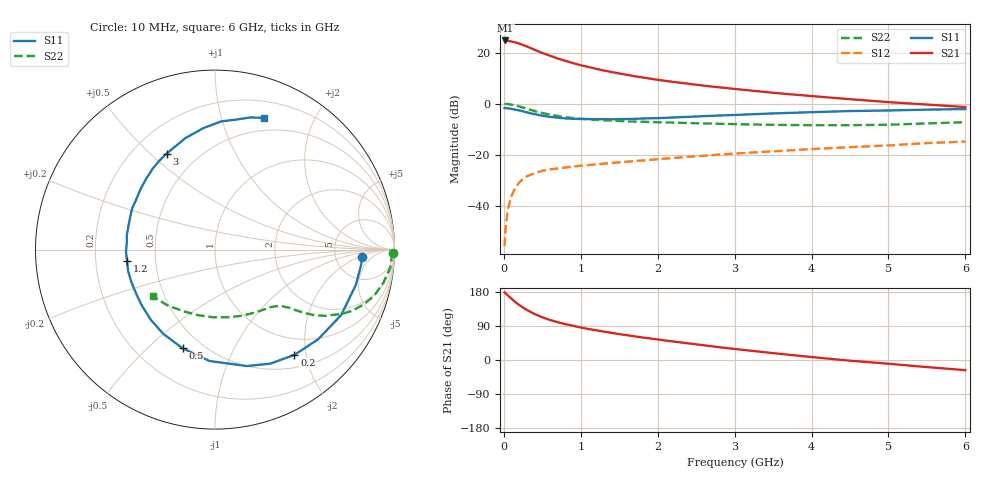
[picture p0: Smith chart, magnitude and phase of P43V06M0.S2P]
! SIEMENS Small Signal Semiconductors
! BFP182
! Si NPN RF Bipolar Junction Transistor in SOT143
! VCE = 3 V  IC = 6 mA
! Common Emitter S-Parameters:  March  1996
# GHz  S  MA  R  50
!  f  S11  S21  S12  S22
! GHz  MAG  ANG  MAG  ANG  MAG  ANG  MAG  ANG
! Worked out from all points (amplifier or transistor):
!   36 points, 10 MHz to 6 GHz, reference 50 ohm
!   highest |S21| = 24.8 dB at 20 MHz (marker M1)
!   |S21| within 3 dB of that: start of sweep to 349.4 MHz
!   unconditionally stable (mu >= 1): 1.477 GHz to 5.459 GHz
!   at 250 MHz: K = 0.24, MSG = 26.2 dB, |S12| = -29.5 dB
!   at 1.4 GHz: K = 0.98, MSG = 17.9 dB, |S12| = -23.3 dB
!   at 6 GHz: K = 0.93, MSG = 6.8 dB, |S12| = -14.9 dB
!   lowest NFmin = 1.25 dB at 450 MHz
!   S11 on the Smith chart (normalised r, x): 10 MHz: 9.55, -2.24; 200 MHz: 0.70, -1.79; 500 MHz: 0.39, -0.65; 1.2 GHz: 0.34, -0.05; 3 GHz: 0.34, +0.56; 6 GHz: 0.36, +1.38
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0.01  0.8195 -2.7  17.16 178.2  0.0016 78.4  0.9892 -1.1
0.02  0.8191 -5.7  17.35 176.6  0.0032 89.8  0.9848 -2.3
0.05  0.809 -14.1  17.15 170.6  0.0083 85.6  0.9822 -5.8
0.1  0.792 -27.4  16.53 161.7  0.0155 75.0  0.9556 -11.2
0.15  0.7617 -41.0  15.91 152.9  0.0224 69.1  0.9234 -16.2
0.2  0.7346 -53.0  15.06 145.1  0.0284 64.0  0.881 -20.4
0.25  0.7064 -64.1  14.07 138.1  0.0334 58.9  0.8376 -24.0
0.3  0.6724 -74.8  13.21 132.0  0.0377 55.3  0.7919 -26.9
0.4  0.6212 -92.9  11.39 121.2  0.0432 48.7  0.715 -31.1
0.5  0.5783 -108.2  9.843 112.7  0.0482 44.6  0.6555 -33.7
0.6  0.551 -121.4  8.719 105.6  0.0513 41.2  0.6086 -35.4
0.7  0.53 -132.5  7.665 99.8  0.0535 39.8  0.5709 -36.6
0.8  0.5131 -142.6  6.92 94.5  0.0558 38.3  0.5426 -37.6
1.1  0.4985 -166.2  5.229 81.8  0.0624 36.6  0.4922 -40.0
1.2  0.4945 -172.9  4.816 78.4  0.0642 36.2  0.4808 -41.0
1.7  0.5033 161.0  3.445 62.5  0.0746 36.2  0.4439 -46.4
2.2  0.5344 141.0  2.671 48.8  0.0857 35.9  0.4241 -53.6
3  0.5992 116.7  1.945 29.2  0.1048 33.4  0.3969 -68.5
3.5  0.6426 104.9  1.633 18.1  0.116 30.9  0.3835 -79.5
4.5  0.7153 87.2  1.222 -1.8  0.14 25.3  0.3775 -104.6
5.5  0.7623 75.0  0.959 -18.7  0.1682 19.5  0.4091 -130.8
6  0.7835 69.4  0.858 -26.8  0.1801 15.0  0.4332 -143.3
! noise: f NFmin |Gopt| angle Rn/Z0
0.45  1.25  0.25  39  0.3
0.9  1.4  0.25  78  0.23
1.8  1.95  0.21  151  0.2
